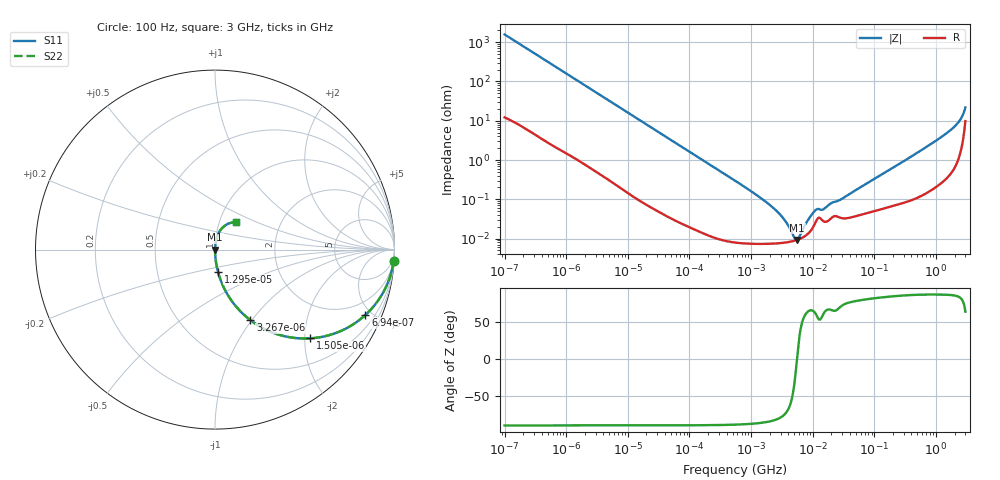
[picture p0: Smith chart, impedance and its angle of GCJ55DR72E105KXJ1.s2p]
!Murata Part Number: GCJ55DR72E105KXJ1
!These Parameters are Measured in Series Mode Connection
!Data Generated on Mar 13, 2026
!  o--ll--o
!Port1  Port2
!  o------o
!Operation Temp=25[degC], DC Bias Voltage=0[V]
!Freq. Start=100[Hz] Stop=3[GHz] 401[Steps]
# Hz S RI R 50
!Freq.(Hz) S11(Real) S11(Imag) S21(Real) S21(Imag) S12(Real) S12(Imag) S22(Real) S22(Imag)
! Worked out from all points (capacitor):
!   401 points, 100 Hz to 3 GHz, reference 50 ohm
!   read as one part in series: C = 1.01 uF near 109 Hz
!   lowest |Z| = 9.26 mohm at 5.597 MHz (marker M1)
!   series resonance near 5.546 MHz, so ESL is about 820 pH
!   S11 on the Smith chart (normalised r, x): 100 Hz: 1, -32; 694 Hz: 1.04, -4.59; 1.505 kHz: 1.02, -2.13; 3.267 kHz: 1.01, -0.98; 12.95 kHz: 1.00, -0.25; 3 GHz: 1.20, +0.39
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100  0.9955 -0.0632  0.0045 0.0632  0.0045 0.0632  0.9955 -0.0632
334  0.9561 -0.2007  0.0439 0.2007  0.0439 0.2007  0.9561 -0.2007
694  0.8384 -0.3636  0.1616 0.3636  0.1616 0.3636  0.8384 -0.3636
1505  0.5304 -0.4943  0.4696 0.4943  0.4696 0.4943  0.5304 -0.4943
1788  0.446 -0.4923  0.554 0.4923  0.554 0.4923  0.446 -0.4923
3267  0.1975 -0.3934  0.8025 0.3934  0.8025 0.3934  0.1975 -0.3934
5968  0.0702 -0.251  0.9298 0.251  0.9298 0.251  0.0702 -0.251
12951  0.0165 -0.123  0.9835 0.123  0.9835 0.123  0.0165 -0.123
31977  0.00306 -0.0508  0.9969 0.0508  0.9969 0.0508  0.00306 -0.0508
547723  8.79e-05 -0.00298  0.9999 0.00298  0.9999 0.00298  8.79e-05 -0.00298
2470636  7.5e-05 -0.000537  0.9999 0.000537  0.9999 0.000537  7.5e-05 -0.000537
3639519  7.93e-05 -0.00026  0.9999 0.00026  0.9999 0.00026  7.93e-05 -0.00026
4919190  8.7e-05 -7.24e-05  0.9999 7.24e-05  0.9999 7.24e-05  8.7e-05 -7.24e-05
5597215  9.24e-05 5.7e-06  0.9999 -5.7e-06  0.9999 -5.7e-06  9.24e-05 5.7e-06
6100390  9.72e-05 5.82e-05  0.9999 -5.82e-05  0.9999 -5.82e-05  9.72e-05 5.82e-05
9794414  0.000179 0.000381  0.9998 -0.000381  0.9998 -0.000381  0.000179 0.000381
1.163455e7  0.000299 0.000471  0.9997 -0.000471  0.9997 -0.000471  0.000299 0.000471
1.506283e7  0.000273 0.000491  0.9997 -0.000491  0.9997 -0.000491  0.000273 0.000491
1.751444e8  0.000667 0.00552  0.9993 -0.00552  0.9993 -0.00552  0.000667 0.00552
1.573002e9  0.00631 0.0508  0.9937 -0.0508  0.9937 -0.0508  0.00631 0.0508
2.317205e9  0.0185 0.0886  0.9815 -0.0886  0.9815 -0.0886  0.0185 0.0886
3e9  0.117 0.1562  0.883 -0.1562  0.883 -0.1562  0.117 0.1562
